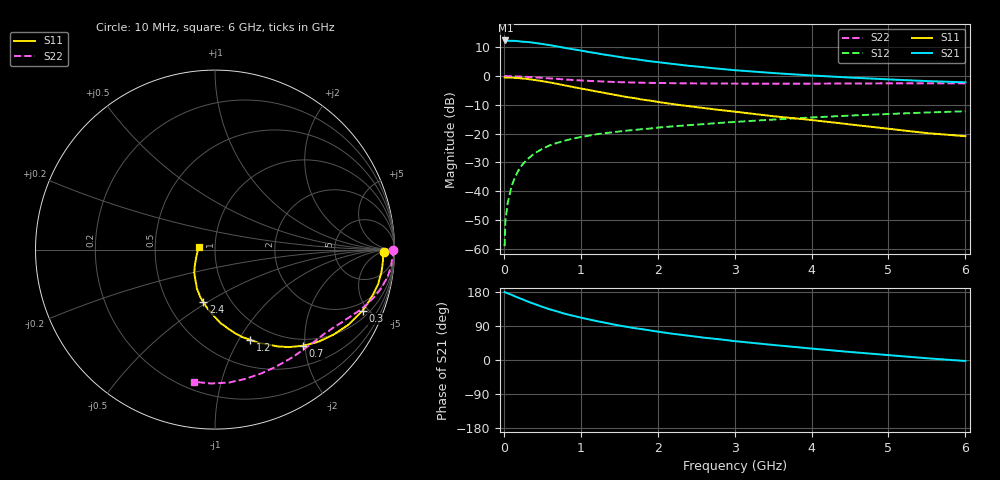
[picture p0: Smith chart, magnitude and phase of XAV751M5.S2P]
! SIEMENS Discrete & RF Semiconductors
! BFY180
! Si NPN RF Bipolar Junction Transistor in MICRO-X
! VCE = 0.75 V  IC = 1.5 mA
! Common Emitter S-Parameters:  May  1997
# GHz  S  MA  R  50
!  f  S11  S21  S12  S22
! GHz  MAG  ANG  MAG  ANG  MAG  ANG  MAG  ANG
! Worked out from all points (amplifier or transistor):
!   36 points, 10 MHz to 6 GHz, reference 50 ohm
!   highest |S21| = 12.4 dB at 20 MHz (marker M1)
!   |S21| within 3 dB of that: start of sweep to 888.9 MHz
!   unconditionally stable (mu >= 1): 1.818 GHz to end of sweep
!   at 250 MHz: K = 0.17, MSG = 21.2 dB, |S12| = -30.5 dB
!   at 1.4 GHz: K = 0.86, MSG = 13.3 dB, |S12| = -19.6 dB
!   at 6 GHz: K = 1.23, MAG = 2.1 dB, |S12| = -12.3 dB
!   S11 on the Smith chart (normalised r, x): 10 MHz: 32, -7; 300 MHz: 1.41, -4.61; 700 MHz: 0.86, -1.96; 1.2 GHz: 0.79, -1.12; 2.4 GHz: 0.75, -0.48; 6 GHz: 0.84, +0.03
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0.01  0.9418 -0.7  4.078 179.5  0.0011 88.4  0.9911 -0.2
0.02  0.9355 -1.5  4.15 178.3  0.003 86.6  0.9999 -0.7
0.05  0.9382 -3.7  4.101 176.0  0.0062 81.9  0.9913 -1.8
0.1  0.9359 -7.5  4.09 171.9  0.0121 84.9  0.9872 -3.6
0.2  0.9182 -15.1  4.01 163.4  0.024 79.9  0.9795 -7.1
0.3  0.8898 -22.5  3.914 155.2  0.0351 75.2  0.965 -10.4
0.4  0.8531 -29.4  3.768 147.6  0.0453 70.8  0.9483 -13.5
0.5  0.8126 -35.7  3.604 140.4  0.0541 66.6  0.9276 -16.3
0.6  0.7718 -41.7  3.435 133.5  0.0625 63.3  0.9081 -18.8
0.7  0.7264 -47.5  3.255 127.8  0.0692 59.9  0.889 -21.0
0.8  0.6829 -52.7  3.069 121.6  0.0757 57.4  0.8705 -23.2
1.1  0.5725 -65.1  2.618 107.4  0.0915 51.1  0.8226 -28.5
1.2  0.5402 -68.6  2.495 102.9  0.0969 49.2  0.8121 -30.2
1.5  0.4553 -79.4  2.149 90.9  0.1087 45.3  0.783 -34.7
1.7  0.4114 -85.6  1.975 84.1  0.1155 43.4  0.7685 -37.5
2.2  0.3241 -98.2  1.621 69.1  0.1333 39.2  0.7504 -44.7
2.4  0.2991 -102.7  1.506 64.1  0.1397 37.7  0.7449 -47.5
3  0.2402 -114.7  1.262 49.8  0.1588 33.4  0.7376 -55.7
3.5  0.2001 -123.1  1.126 39.7  0.1748 29.9  0.7355 -62.7
4.5  0.144 -141.5  0.94 21.2  0.2052 21.8  0.7402 -76.8
5.5  0.1016 -169.1  0.816 4.6  0.2319 13.2  0.7463 -91.7
6  0.0899 169.8  0.776 -2.6  0.2437 8.6  0.7454 -99.0
